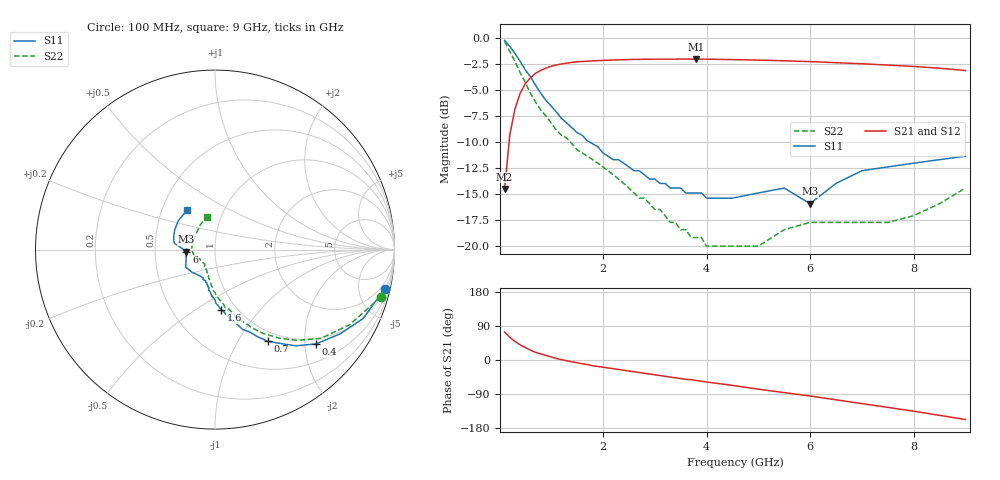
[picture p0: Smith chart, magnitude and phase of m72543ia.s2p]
!  MGA-72543 S PARAMETERS
!  Vd=3V  Id=0 mA Vc=3V  LAST UPDATED 01-27-99
# ghz s ma r 50
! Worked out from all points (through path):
!   50 points, 100 MHz to 9 GHz, reference 50 ohm
!   highest |S21| = -2.05 dB at 3.8 GHz (marker M1); lowest = -14.5 dB at 100 MHz (marker M2)
!   group delay of S21, straight-line fit = 61.4 ps
!   lowest |S11| = -15.9 dB at 6 GHz (marker M3), VSWR 1.38, Z = 36.2 - j0.83 ohm
!   |S11| at or under -10 dB: 1.737 GHz to end of sweep
!   |S22| runs from -20.0 to -0.4 dB; largest |S21 - S12| = 0.014
!   S11 on the Smith chart (normalised r, x): 100 MHz: 1.17, -8.62; 400 MHz: 0.87, -2.25; 700 MHz: 0.86, -1.35; 1.6 GHz: 0.85, -0.65; 6 GHz: 0.72, -0.02; 9 GHz: 0.67, +0.32
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0.1  0.97 -13.0  0.188 74.0  0.188 74.0  0.96 -16.0
0.2  0.91 -25.0  0.341 60.0  0.342 60.0  0.86 -29.0
0.3  0.84 -34.0  0.456 49.0  0.456 49.0  0.77 -40.0
0.4  0.77 -43.0  0.541 40.0  0.541 40.0  0.68 -48.0
0.5  0.7 -50.0  0.602 33.0  0.602 33.0  0.61 -54.0
0.6  0.65 -54.0  0.643 26.0  0.643 26.0  0.54 -60.0
0.7  0.59 -60.0  0.675 20.0  0.675 21.0  0.49 -64.0
1  0.47 -71.0  0.73 8.0  0.73 8.0  0.39 -73.0
1.6  0.34 -84.0  0.769 -10.0  0.769 -10.0  0.28 -85.0
2.3  0.26 -94.0  0.783 -25.0  0.783 -25.0  0.21 -94.0
3.1  0.2 -102.0  0.789 -41.0  0.789 -41.0  0.15 -106.0
3.3  0.19 -104.0  0.789 -45.0  0.788 -45.0  0.13 -110.0
3.8  0.18 -110.0  0.79 -54.0  0.789 -54.0  0.11 -120.0
3.9  0.18 -112.0  0.789 -56.0  0.789 -56.0  0.11 -122.0
4  0.17 -113.0  0.789 -58.0  0.789 -58.0  0.1 -124.0
5  0.18 -136.0  0.781 -77.0  0.781 -77.0  0.1 -150.0
5.5  0.19 -149.0  0.775 -86.0  0.775 -86.0  0.12 -161.0
6  0.16 -176.0  0.768 -95.0  0.768 -95.0  0.13 -178.0
6.5  0.2 175.0  0.759 -105.0  0.759 -105.0  0.13 170.0
7  0.23 171.0  0.75 -115.0  0.75 -115.0  0.13 160.0
8  0.25 154.0  0.728 -135.0  0.728 -135.0  0.14 137.0
9  0.27 125.0  0.696 -157.0  0.696 -157.0  0.19 104.0
